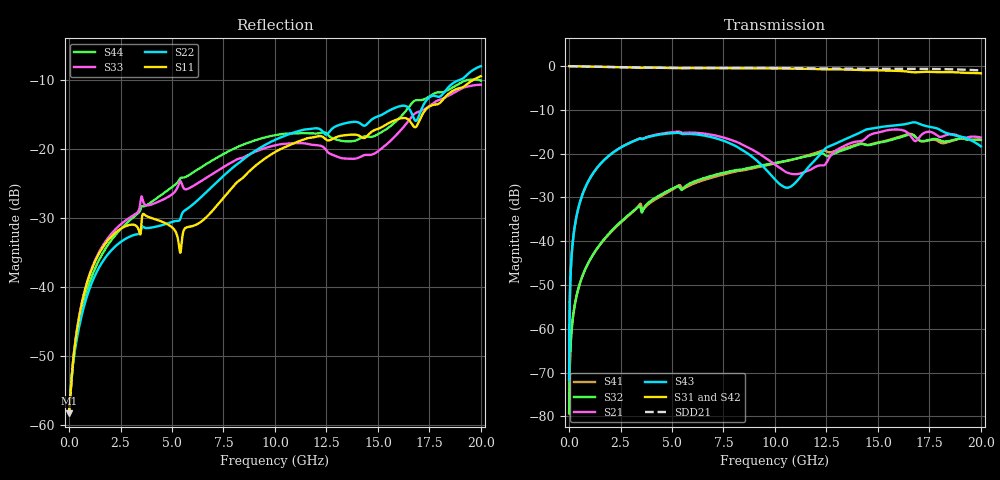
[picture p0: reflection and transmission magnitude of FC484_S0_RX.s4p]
! MPF300XT FC484 S-parameter file
! Microsemi Corporation (c) 2018
!Initial ver: Mar 8, 2018
! Exported from HFSS 3D Layout Design 2017.2.0
! Port[1] = BGA.M21.SERDES_0_RX0_N
! Port[2] = BGA.M22.SERDES_0_RX0_P
! Port[3] = DIE1.544.SERDES_0_RX0_N
! Port[4] = DIE1.545.SERDES_0_RX0_P
# GHz S MA R 50
! freq  S11mag  S11ang  S12mag  S12ang  S13mag  S13ang  S14mag  S14ang
!  S21mag  S21ang  S22mag  S22ang  S23mag  S23ang  S24mag  S24ang
!  S31mag  S31ang  S32mag  S32ang  S33mag  S33ang  S34mag  S34ang
!  S41mag  S41ang  S42mag  S42ang  S43mag  S43ang  S44mag  S44ang
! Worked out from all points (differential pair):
!   4999 points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, 4.001 MHz to 20 GHz, reference 50 ohm
!   strongest paths, dB at 4.001 MHz, 5.001 GHz, 10 GHz, 15 GHz, 20 GHz:
!     S31: 0.0, -0.4, -0.5, -1.0, -1.6
!     S42: 0.0, -0.4, -0.5, -1.0, -2.3
!     S43: -71.7, -15.3, -25.9, -14.0, -18.3
!     S21: -71.7, -15.1, -22.5, -15.2, -16.3
!     S32: -79.3, -28.0, -22.1, -17.5, -16.9
!     S41: -79.3, -28.3, -22.3, -17.4, -16.7
!   taken as a pair (ports 1,2 in; 3,4 out), SDD21 dB: 0.0, -0.4, -0.4, -0.6, -1.0
!   lowest |S11| = -58.3 dB at 4.001 MHz (marker M1), VSWR 1.00, Z = 50.1 + j0.00674 ohm
!   |S11| at or under -10 dB: start of sweep to 19.62 GHz
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0.0040008  0.00122 3.2  0.0002602 67.8  0.9988 -0.1  0.0001086 -153.0
           0.0002602 67.8  0.00122 3.6  0.0001086 -153.0  0.9988 -0.1
           0.9988 -0.1  0.0001086 -153.0  0.00122 3.2  0.0002602 67.8
           0.0001086 -153.0  0.9988 -0.1  0.0002602 67.8  0.00122 3.7
0.1720344  0.002656 -14.4  0.009312 84.5  0.9966 -3.3  0.001258 -108.3
           0.009312 84.5  0.002591 -5.0  0.001258 -108.2  0.9966 -3.3
           0.9966 -3.3  0.001258 -108.2  0.002667 -13.1  0.009313 84.2
           0.001258 -108.3  0.9966 -3.3  0.009313 84.2  0.002643 -3.8
0.560112  0.006904 -61.6  0.02949 78.8  0.9927 -10.3  0.003492 -106.8
          0.02949 78.8  0.005757 -54.1  0.003496 -106.3  0.9927 -10.4
          0.9927 -10.3  0.003496 -106.3  0.006982 -56.6  0.02948 77.9
          0.003492 -106.8  0.9927 -10.4  0.02948 77.9  0.006176 -46.6
2.916583  0.02816 -141.5  0.1325 40.0  0.9709 -52.2  0.01984 -134.9
          0.1325 40.0  0.0231 -150.3  0.02027 -134.4  0.9711 -52.3
          0.9709 -52.2  0.02027 -134.4  0.03164 -104.6  0.1317 35.3
          0.01984 -134.9  0.9711 -52.3  0.1317 35.3  0.03016 -93.7
10.35407  0.1013 -25.1  0.06559 -35.9  0.9399 178.6  0.08073 83.1
          0.06559 -35.9  0.1224 -17.0  0.08145 82.4  0.9364 177.9
          0.9399 178.6  0.08145 82.4  0.1088 -159.7  0.04289 -161.3
          0.08073 83.1  0.9364 177.9  0.04289 -161.3  0.1286 -168.0
15.03501  0.1405 -51.9  0.1749 -13.1  0.8958 96.1  0.135 -10.1
          0.1749 -13.1  0.1728 -48.4  0.1333 -6.9  0.886 94.6
          0.8958 96.1  0.1333 -6.9  0.09717 41.9  0.1997 11.2
          0.135 -10.1  0.886 94.6  0.1997 11.2  0.1291 37.2
20  0.3369 -66.3  0.1533 -79.5  0.8281 10.3  0.1463 -118.4
    0.1533 -79.5  0.3982 -71.7  0.1431 -119.7  0.7652 7.7
    0.8281 10.3  0.1431 -119.7  0.2922 -105.9  0.1212 -142.9
    0.1463 -118.4  0.7652 7.7  0.1212 -142.9  0.3129 -119.2
